[IBIS Ver]   3.2
[File Name]   sprm143.ibs
[File Rev]   0.6
[Date]   July 31, 2008
[Source]   IBIS Model Generated from PACED 4.51D
[Disclaimer]   Please be aware that in the absence of a written agreement
|   Texas Instruments(TI) assumes no liability for:
|   (1) The accuracy of the IBIS models provided to your company
|   (2) The proper functioning of these Models in your design
|   or for any resulting applications; or
|   (3)Infringement of patents, copyrights or intellectual
|   property rights resulting from your use of these models.
|   TI provides IBIS Models as a service to our customers and
|   therefore reserves the right to limit distribution of the
|   Models.
[Copyright]   Property of Texas Instruments Incorporated.
|   Unauthorized reproduction and/or distribution is strictly.
|   prohibited.
|   This product is protected under copyright law and trade
|   secret law as an unpublished work.
|   Created 2002,(C) Copyright 2002,
|   Texas Instruments Incorporated., All Rights Reserved.
|   These commodities are under the U.S.
|   Government distribution license control. As such,they are
|   not to be re-exported without the prior approval of the U.S.
|   Department of Commerce.
[Notes]   Revision History
|   0.4  Updated CLKOUT3 buffer to reflect silicon revision 2.0
|   for C6713B PYP device.
|   0.5 Added OUK831PE1001 buffer definition.
|   0.6 Fixed swapped min/max values for UOS335PE1001 C_comp
[Component]   c6713B_PYP
[Manufacturer]   Texas Instruments
[Package]
| Variable   Typ   Min   Max
R_pkg   0.1327   0.1187   0.1442
L_pkg   2.801e-09   2.511e-09   3.057e-09
C_pkg   2.69e-13   2.056e-13   3.082e-13
[Pin] signal_name   model_name   R_pin   L_pin   C_pin
204  CLKIN   IDH091PE1001   1.80E-01   8.61E-09   1.87E-12
82   CLKOUT2/GP2   IDH091UOS335PE1001   1.76E-01   7.19E-09   1.51E-12
184  CLKOUT3   OUK831PE1001   1.77E-01   7.15E-09   1.50E-12
205  CLKMODE0   IDH091PS1001   1.81E-01   8.75E-09   1.90E-12
192  TMS   IDH091PS1001   1.76E-01   7.51E-09   1.61E-12
187  TDO   OUK831PS1001   1.76E-01   7.23E-09   1.55E-12
191  TDI   IDH091PS1001   1.75E-01   7.44E-09   1.57E-12
193  TCK   IDH091PS1001   1.76E-01   7.58E-09   1.63E-12
197  TRSTz   IDH091PE1001   1.80E-01   7.95E-09   1.70E-12
185  EMU1   IDH091OUK831PS1001   1.77E-01   7.18E-09   1.54E-12
186  EMU0   IDH091OUK831PS1001   1.76E-01   7.18E-09   1.54E-12
176  RESETz   IDG091PS1001   1.76E-01   7.33E-09   1.58E-12
175  NMI   IDH091PE1001   1.76E-01   7.39E-09   1.59E-12
7   GP7   IDH091OUK831PS1001   1.71E-01   8.22E-09   1.76E-12
2   GP6   IDH091OUK831PS1001   1.69E-01   8.72E-09   1.89E-12
6   GP5/AMUTEIN0   IDH091OUK831PS1001   1.71E-01   8.31E-09   1.78E-12
1   GP4/AMUTEIN1   IDH091OUK831PS1001   1.72E-01   9.01E-09   1.52E-12
135  HINTz/GP1   IDH091OUK831PS1001   1.63E-01   6.96E-09   1.53E-12
144  HCNTRL1/AXR1_1   IDH091OUK831PS1001   1.73E-01   7.73E-09   1.64E-12
146  HCNTRL0/AXR1_3   IDH091OUK831PS1001   1.76E-01   7.96E-09   1.67E-12
139  HHWIL/AFSR1   IDH091OUK831PS1001   1.65E-01   7.23E-09   1.56E-12
143  HRW/AXR1_0   IDH091OUK831PS1001   1.72E-01   7.64E-09   1.64E-12
174  HD15/GP15   IDH091OUK831PS1001   1.76E-01   7.46E-09   1.58E-12
173  HD14/GP14   IDH091OUK831PS1001   1.76E-01   7.52E-09   1.60E-12
172  HD13/GP13   IDH091OUK831PS1001   1.77E-01   7.60E-09   1.63E-12
168  HD12/GP12   IDH091OUK831PS1001   1.81E-01   7.98E-09   1.67E-12
167  HD11/GP11   IDH091OUK831PS1001   1.84E-01   8.11E-09   1.67E-12
166  HD10/GP10   IDH091OUK831PS1001   1.82E-01   8.15E-09   1.72E-12
165  HD9/GP9   IDH091OUK831PS1001   1.83E-01   8.25E-09   1.76E-12
160  HD8/GP8   IDH091OUK831PS1001   1.82E-01   8.76E-09   1.87E-12
164  HD7/GP3   IDH091OUK831PS1001   1.83E-01   8.36E-09   1.79E-12
161  HD6/AHCLKR1   IDH091OUK831PS1001   1.84E-01   8.69E-09   1.85E-12
159  HD5/AHCLKX1   IDH091OUK831PS1001   1.83E-01   8.87E-09   1.89E-12
156  HD4/GP0   IDH091OUK831PE1001   1.81E-01   9.23E-09   1.54E-12
154  HD3/AMUTE1   IDH091OUK831PS1001   1.78E-01   8.80E-09   1.88E-12
155  HD2/AFSX1   IDH091OUK831PS1001   1.79E-01   8.93E-09   1.90E-12
152  HD1/AXR1_7   IDH091OUK831PS1001   1.83E-01   8.68E-09   1.84E-12
147  HD0/AXR1_4   IDH091OUK831PS1001   1.76E-01   8.04E-09   1.70E-12
153  HASz/ACLKX1   IDH091OUK831PS1001   1.81E-01   8.76E-09   1.86E-12
145  HCSz/AXR1_2   IDH091OUK831PS1001   1.74E-01   7.82E-09   1.67E-12
151  HDS1z/AXR1_6   IDH091OUK831PS1001   1.83E-01   8.57E-09   1.84E-12
150  HDS2z/AXR1_5   IDH091OUK831PS1001   1.81E-01   8.42E-09   1.83E-12
140  HRDYz/ACLKR1   IDH091OUK831PE1001   1.67E-01   7.32E-09   1.60E-12
57   CE3z   IDH091OUK831PS1001   1.90E-01   8.82E-09   1.88E-12
61   CE2z   IDH091OUK831PS1001   1.85E-01   8.31E-09   1.77E-12
103  CE1z   IDH091OUK831PS1001   1.92E-01   9.21E-09   1.93E-12
102  CE0z   IDH091OUK831PS1001   1.90E-01   9.04E-09   1.92E-12
108  BE1z   IDH091OUK831PS1001   1.67E-01   8.44E-09   1.86E-12
110  BE0z   IDH091OUK831PS1001   1.66E-01   8.20E-09   1.78E-12
137  HOLDAz   IDH091OUK831PS1001   1.65E-01   7.10E-09   1.56E-12
138  HOLDz   IDH091OUK831PS1001   1.66E-01   7.19E-09   1.54E-12
136  BUSREQ   IDH091OUK831PS1001   1.64E-01   7.02E-09   1.54E-12
78   ECLKIN   IDH091PE1001   1.77E-01   7.16E-09   1.35E-12
77   ECLKOUT   UOS335PE1001   1.77E-01   7.16E-09   1.52E-12
79   SDCASz   IDH091OUK831PS1001   1.77E-01   7.14E-09   1.37E-12
75   SDRASz   IDH091OUK831PS1001   1.77E-01   7.20E-09   1.52E-12
83   SDWEz   IDH091OUK831PS1001   1.76E-01   7.24E-09   1.52E-12
56   ARDY   IDH091OUK831PS1001   1.92E-01   8.97E-09   1.87E-12
109  EA21   IDH091OUK831PS1001   1.65E-01   8.30E-09   1.82E-12
101  EA20   IDH091OUK831PS1001   1.91E-01   8.96E-09   1.90E-12
100  EA19   IDH091OUK831PS1001   1.89E-01   8.81E-09   1.89E-12
95   EA18   IDH091OUK831PS1001   1.85E-01   8.23E-09   1.73E-12
99   EA17   IDH091OUK831PS1001   1.88E-01   8.67E-09   1.86E-12
92   EA16   IDH091OUK831PS1001   1.81E-01   7.89E-09   1.68E-12
94   EA15   IDH091OUK831PS1001   1.84E-01   8.12E-09   1.70E-12
90   EA14   IDH091OUK831PS1001   1.79E-01   7.70E-09   1.65E-12
91   EA13   IDH091OUK831PS1001   1.80E-01   7.79E-09   1.67E-12
93   EA12   IDH091OUK831PS1001   1.83E-01   8.00E-09   1.70E-12
86   EA11   IDH091OUK831PS1001   1.76E-01   7.39E-09   1.59E-12
76   EA10   IDH091OUK831PS1001   1.78E-01   7.21E-09   1.52E-12
74   EA9   IDH091OUK831PS1001   1.77E-01   7.25E-09   1.55E-12
71   EA8   IDH091OUK831PS1001   1.77E-01   7.43E-09   1.56E-12
70   EA7   IDH091OUK831PS1001   1.77E-01   7.47E-09   1.57E-12
69   EA6   IDH091OUK831PS1001   1.77E-01   7.54E-09   1.62E-12
68   EA5   IDH091OUK831PS1001   1.78E-01   7.62E-09   1.63E-12
64   EA4   IDH091OUK831PS1001   1.83E-01   8.02E-09   1.66E-12
63   EA3   IDH091OUK831PS1001   1.84E-01   8.12E-09   1.68E-12
62   EA2   IDH091OUK831PS1001   1.85E-01   8.20E-09   1.75E-12
112  ED15   IDH091OUK831PS1001   1.65E-01   7.98E-09   1.75E-12
113  ED14   IDH091OUK831PS1001   1.66E-01   7.90E-09   1.73E-12
111  ED13   IDH091OUK831PS1001   1.66E-01   8.10E-09   1.77E-12
118  ED12   IDH091OUK831PS1001   1.61E-01   7.39E-09   1.63E-12
117  ED11   IDH091OUK831PS1001   1.62E-01   7.48E-09   1.65E-12
120  ED10   IDH091OUK831PS1001   1.60E-01   7.25E-09   1.56E-12
119  ED9   IDH091OUK831PS1001   1.60E-01   7.30E-09   1.60E-12
123  ED8   IDH091OUK831PS1001   1.60E-01   7.04E-09   1.56E-12
122  ED7   IDH091OUK831PS1001   1.60E-01   7.11E-09   1.56E-12
121  ED6   IDH091OUK831PS1001   1.60E-01   7.18E-09   1.55E-12
128  ED5   IDH091OUK831PS1001   1.61E-01   6.86E-09   1.51E-12
127  ED4   IDH091OUK831PS1001   1.60E-01   6.84E-09   1.52E-12
129  ED3   IDH091OUK831PS1001   1.61E-01   6.81E-09   1.50E-12
130  ED2   IDH091OUK831PS1001   1.62E-01   6.82E-09   1.34E-12
131  ED1   IDH091OUK831PS1001   1.61E-01   6.81E-09   1.34E-12
132  ED0   IDH091OUK831PS1001   1.62E-01   6.81E-09   1.52E-12
13   TOUT1/AXR0_4   IDH091OUK831PE1001   1.74E-01   7.74E-09   1.68E-12
12   TINP1/AHCLKX0   IDH091OUK831PE1001   1.76E-01   7.87E-09   1.68E-12
18   TOUT0/AXR0_2   IDH091OUK831PE1001   1.66E-01   7.24E-09   1.59E-12
17   TINP0/AXR0_3   IDH091OUK831PE1001   1.68E-01   7.33E-09   1.61E-12
8   CLKS1/SCL1   IDG091UOS205   1.73E-01   8.16E-09   1.72E-12
36   CLKR1/AXR0_6   IDH091OUK831PE1001   1.62E-01   7.21E-09   1.60E-12
33   CLKX1/AMUTE0   IDH091OUK831PE1001   1.61E-01   7.00E-09   1.55E-12
37   DR1/SDA1   IDG091UOS205   1.63E-01   7.30E-09   1.62E-12
32   DX1/AXR0_5   IDH091OUK831PS1001   1.60E-01   6.94E-09   1.54E-12
38   FSR1/AXR0_7   IDH091OUK831PE1001   1.64E-01   7.39E-09   1.63E-12
31   FSX1   IDH091OUK831PE1001   1.60E-01   6.89E-09   1.53E-12
28   CLKS0/AHCLKR0   IDH091OUK831PE1001   1.61E-01   6.79E-09   1.52E-12
19   CLKR0/ACLKR0   IDH091OUK831PE1001   1.65E-01   7.16E-09   1.58E-12
16   CLKX0/ACLKX0   IDH091OUK831PE1001   1.69E-01   7.44E-09   1.61E-12
27   DR0/AXR0_0   IDH091OUK831PS1001   1.61E-01   6.79E-09   1.37E-12
20   DX0/AXR0_1   IDH091OUK831PS1001   1.64E-01   7.08E-09   1.57E-12
24   FSR0/AFSR0   IDH091OUK831PE1001   1.62E-01   6.87E-09   1.53E-12
21   FSX0/AFSX0   IDH091OUK831PE1001   1.63E-01   7.00E-09   1.55E-12
41   SCL0   IDG091UOS205   1.69E-01   7.72E-09   1.69E-12
42   SDA0   IDG091UOS205   1.72E-01   7.85E-09   1.69E-12
| End of package information
| Component   IDG091PS1001
[Component]   IDG091PS1001
[Manufacturer]   Texas Instruments
[Package]
|   typ   min   max
R_pkg   0   0   0
L_pkg   0   0   0
C_pkg   0   0   0
[Pin]   signal_name   model_name   R_pin   L_pin   C_pin
   1   A   IDG091PS1001   0   0   0
| Component   IDG091UOS205
[Component]   IDG091UOS205
[Manufacturer]   Texas Instruments
[Package]
|   typ   min   max
R_pkg   0   0   0
L_pkg   0   0   0
C_pkg   0   0   0
[Pin]   signal_name   model_name   R_pin   L_pin   C_pin
   1   Y   IDG091UOS205   0   0   0
| Component   IDH091OUK831PE1001
[Component]   IDH091OUK831PE1001
[Manufacturer]   Texas Instruments
[Package]
|   typ   min   max
R_pkg   0   0   0
L_pkg   0   0   0
C_pkg   0   0   0
[Pin]   signal_name   model_name   R_pin   L_pin   C_pin
   1   Y  IDH091OUK831PE1001   0   0   0
| Component   IDH091OUK831PS1001
[Component]   IDH091OUK831PS1001
[Manufacturer]   Texas Instruments
[Package]
|   typ   min   max
R_pkg   0   0   0
L_pkg   0   0   0
C_pkg   0   0   0
[Pin]   signal_name   model_name   R_pin   L_pin   C_pin
   1   Y  IDH091OUK831PS1001   0   0   0
| Component   IDH091PE1001
[Component]   IDH091PE1001
[Manufacturer]   Texas Instruments
[Package]
|   typ   min   max
R_pkg   0   0   0
L_pkg   0   0   0
C_pkg   0   0   0
[Pin]   signal_name   model_name   R_pin   L_pin   C_pin
   1   A   IDH091PE1001   0   0   0
| Component   IDH091PS1001
[Component]   IDH091PS1001
[Manufacturer]   Texas Instruments
[Package]
|   typ   min   max
R_pkg   0   0   0
L_pkg   0   0   0
C_pkg   0   0   0
[Pin]   signal_name   model_name   R_pin   L_pin   C_pin
   1   A   IDH091PS1001   0   0   0
| Component   IDH091UOS335PE1001
[Component]   IDH091UOS335PE1001
[Manufacturer]   Texas Instruments
[Package]
|   typ   min   max
R_pkg   0   0   0
L_pkg   0   0   0
C_pkg   0   0   0
[Pin]   signal_name   model_name   R_pin   L_pin   C_pin
   1   Y  IDH091UOS335PE1001   0   0   0
| Component   OUK831PS1001
[Component]   OUK831PS1001
[Manufacturer]   Texas Instruments
[Package]
|   typ   min   max
R_pkg   0   0   0
L_pkg   0   0   0
C_pkg   0   0   0
[Pin]   signal_name   model_name   R_pin   L_pin   C_pin
   1   Y   OUK831PS1001   0   0   0
| Component   UOS335PE1001
[Component]   UOS335PE1001
[Manufacturer]   Texas Instruments
[Package]
|   typ   min   max
R_pkg   0   0   0
L_pkg   0   0   0
C_pkg   0   0   0
[Pin]   signal_name   model_name   R_pin   L_pin   C_pin
   1   Y   UOS335PE1001   0   0   0
| Component   OUK831PE1001
[Component]   OUK831PE1001
[Manufacturer]   Texas Instruments
[Package]
|   typ   min   max
R_pkg   0   0   0
L_pkg   0   0   0
C_pkg   0   0   0
[Pin]   signal_name   model_name   R_pin   L_pin   C_pin
   1   Y   OUK831PE1001   0   0   0
| Models and submodels in the file (10): IDG091PS1001 (Input), IDG091UOS205 (I/O_open_drain), IDH091OUK831PE1001 (I/O), IDH091OUK831PS1001 (I/O), IDH091PE1001 (Input), IDH091PS1001 (Input), IDH091UOS335PE1001 (I/O), OUK831PS1001 (3-state), UOS335PE1001 (3-state), OUK831PE1001 (3-state)
